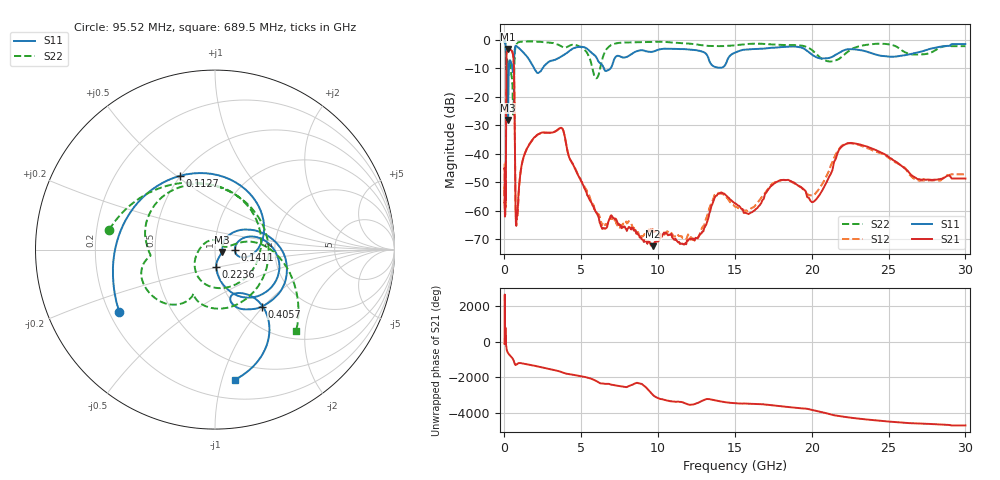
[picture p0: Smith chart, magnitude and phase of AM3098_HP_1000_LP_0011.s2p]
! Date/Time: Thu, Feb 28, 2019 8:39 AM
! Network Analyzer: Agilent Technologies E8364B Rev: A.07.50.67
! Sweep from 0.010 to 30.000 GHz, 1601 Points, Sweep Type: LOG
! Power Supply: 5.022 V, 0.002 A
# Hz S DB R 50
!freq MagS11 AngS11 MagS21 AngS21 MagS12 AngS12 MagS22 AngS22
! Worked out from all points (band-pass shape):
!   1601 points, 10 MHz to 30 GHz, reference 50 ohm
!   highest |S21| = -3.34 dB at 237.5 MHz (marker M1); lowest = -72.4 dB at 9.682 GHz (marker M2)
!   |S21| within 3 dB of the highest: 127.3 MHz to 580 MHz (452.7 MHz wide, 128 % of centre)
!   lowest |S11| = -28.2 dB at 236.3 MHz (marker M3), VSWR 1.08, Z = 53.8 - j1.42 ohm
!   |S11| at or under -10 dB: 198.2 MHz to 288.6 MHz (90.43 MHz wide, 37.2 % of centre); 1.92 GHz to 2.493 GHz (572.7 MHz wide, 26 % of centre); 6.47 GHz to 6.922 GHz (452.7 MHz wide, 6.76 % of centre)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
!   |S22| runs from -26.3 to -0.5 dB; largest |S21 - S12| = 0.011
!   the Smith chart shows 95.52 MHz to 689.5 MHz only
!   S11 on the Smith chart (normalised r, x): 95.52 MHz: 0.24, -0.28; 112.7 MHz: 0.50, +0.52; 141.1 MHz: 1.25, -0.00; 223.6 MHz: 0.99, -0.20; 405.7 MHz: 1.28, -0.98; 689.5 MHz: 0.35, -1.10
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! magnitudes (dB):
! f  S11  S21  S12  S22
! 10 MHz  -0.3  -45.3  -43.4  -0.5
! 38.04 MHz  -0.5  -59.5  -59.1  -0.8
! 82.62 MHz  -2.2  -56.1  -57.9  -2.5
! 95.52 MHz  -3.9  -42.3  -41.3  -4.4
! 112.7 MHz  -6.8  -16.4  -16.4  -10.4
! 141.1 MHz  -19.2  -4.5  -4.5  -11.0
! 144.7 MHz  -18.5  -4.4  -4.3  -10.5
! 223.6 MHz  -20.1  -3.4  -3.4  -8.7
! 236.3 MHz  -28.2  -3.3  -3.3  -8.9
! 237.5 MHz  -28.1  -3.3  -3.3  -8.9
! 405.7 MHz  -7.7  -3.6  -3.6  -10.5
! 550.5 MHz  -11.4  -5.1  -5.1  -24.2
! 627 MHz  -6.4  -12.1  -12.1  -14.6
! 689.5 MHz  -2.7  -42.6  -42.9  -3.9
! 765.9 MHz  -2.2  -64.5  -62.9  -1.6
! 2.084 GHz  -11.4  -33.7  -33.6  -0.7
! 3.742 GHz  -5.8  -31.0  -31.0  -2.5
! 7.926 GHz  -6.1  -66.5  -63.8  -1.0
! 9.682 GHz  -4.2  -72.4  -66.9  -0.9
! 20.2 GHz  -5.9  -56.5  -54.2  -4.6
! 22.67 GHz  -3.4  -36.4  -36.4  -3.2
! 30 GHz  -1.6  -48.7  -47.2  -2.3
